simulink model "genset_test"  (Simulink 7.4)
settings: Solver=ode23t  StartTime=0.0  StopTime=10  RelTol=1e-4
undefined symbols (not defined in the file or in its folder): bits, D1, Delta
libraries: powerlib x25, powerlib_extras x3, dspswit3 x1

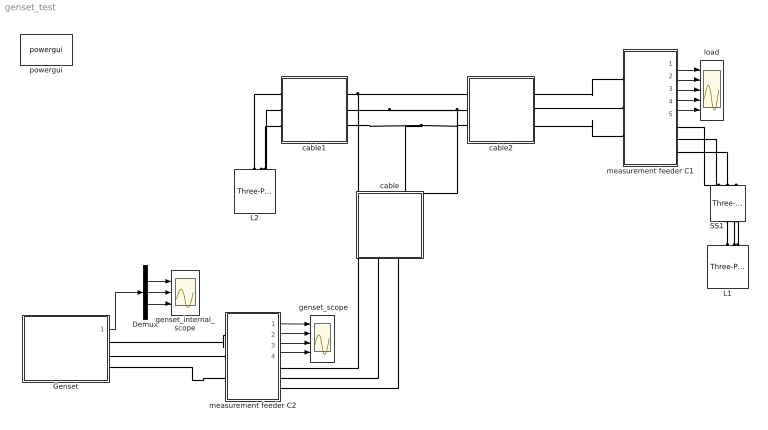
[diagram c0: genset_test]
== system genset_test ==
  " genset_scope" : Scope  NumInputPorts=4
  Demux : Demux  Outputs=3
  Genset : Subsystem
  L1 : powerlib/Elements/Three-Phase Series RLC Load  DialogController=POWERSYS.PowerSysDialog  PhysicalDomain=powersysdomain  SubClassName=unknown  LeftPortType=p1  RightPortType=p1  LConnTagsString=A|B|C  Configuration=Y (grounded)  NominalVoltage=208  NominalFrequency=60  ActivePower=4000  InductivePower=0  CapacitivePower=0  Measurements=None
  L2 : powerlib/Elements/Three-Phase Series RLC Load  DialogController=POWERSYS.PowerSysDialog  PhysicalDomain=powersysdomain  SubClassName=unknown  LeftPortType=p1  RightPortType=p1  LConnTagsString=A|B|C  Configuration=Y (grounded)  NominalVoltage=208  NominalFrequency=60  ActivePower=1897  InductivePower=0  CapacitivePower=0  Measurements=None
  SS1 : powerlib/Elements/Three-Phase Breaker  DialogController=POWERSYS.PowerSysDialog  SystemSampleTime=-1  InitialState=open  SwitchA=on  SwitchB=on  SwitchC=on  SwitchTimes=[3+1/5 7]  External=off  BreakerResistance=.00001  SnubberResistance=1e10  SnubberCapacitance=inf  Measurements=None
  cable : Subsystem  mask{R=.0656, L=.0021, C=345.6}
  cable1 : Subsystem  mask{R=.002657, L=.000641, C=2020}
  cable2 : Subsystem  mask{R=0.0168, L=0.00407, C=336}
  genset_internal_scope : Scope  NumInputPorts=3
  load : Scope  NumInputPorts=5
  measurement feeder C1 : Subsystem
  measurement feeder C2 : Subsystem
  powergui : powerlib/powergui  Priority=1  SystemSampleTime=-1  SimulationMode=Discrete  SampleTime=20e-6  frequency=60  SPID=off  DisableSnubberDevices=off  DisableRonSwitches=off  DisableVfSwitches=off  SwTol=0  Interpol=off  frequencyindice=60  echomessages=off  HookPort=off  DisplayEquations=off  FunctionMessages=off  EnableUseOfTLC=off  x0status=blocks  RestoreLinks=warning  Frange=[0:2:500]  Ylog=off  Xlog=on  ShowGrid=off  save=off  variable=ZData  ZoomFFT=on  StartTime=0.0  cycles=1  DisplayStyle=1  fundamental=60  FreqAxis=off  MaxFrequency=1000  frequencyindicesteady=1  RmsSteady=1  display=off  Ts=0  methode=off
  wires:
  measurement feeder C2/1(Vabc) -> " genset_scope"/1
  measurement feeder C2/2(Iabc) -> " genset_scope"/2
  measurement feeder C2/3(PQ) -> " genset_scope"/3
  measurement feeder C2/4(RMS (V-I)) -> " genset_scope"/4
  measurement feeder C1/5(w) -> load/5
  measurement feeder C1/4(RMS (V-I)) -> load/4
  measurement feeder C1/3(PQ) -> load/3
  measurement feeder C1/2(Iabc) -> load/2
  measurement feeder C1/1(Vabc) -> load/1
  Demux/3 -> genset_internal_scope/3
  Demux/2 -> genset_internal_scope/2
  Demux/1 -> genset_internal_scope/1
  Genset/1(m) -> Demux/1
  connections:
  cable1/RConn2 -- L2/LConn2
  measurement feeder C1/RConn1 -- SS1/LConn1
  measurement feeder C1/RConn2 -- SS1/LConn2
  measurement feeder C1/RConn3 -- SS1/LConn3
  L1/LConn1 -- SS1/RConn1
  L1/LConn2 -- SS1/RConn2
  L1/LConn3 -- SS1/RConn3
  cable1/LConn1 -- cable/RConn1 -- cable2/RConn1
  cable2/RConn2 -- cable/RConn2 -- cable1/LConn2
  cable2/RConn3 -- cable1/LConn3 -- cable/RConn3
  cable2/LConn2 -- measurement feeder C1/LConn2
  measurement feeder C2/LConn1 -- Genset/RConn1
  Genset/RConn3 -- measurement feeder C2/LConn3
  measurement feeder C2/RConn1 -- cable/LConn1
  measurement feeder C2/RConn2 -- cable/LConn2
  measurement feeder C2/RConn3 -- cable/LConn3
  cable1/RConn1 -- L2/LConn1
  L2/LConn3 -- cable1/RConn3
  measurement feeder C1/LConn1 -- cable2/LConn1
  measurement feeder C1/LConn3 -- cable2/LConn3
  Genset/RConn2 -- measurement feeder C2/LConn2

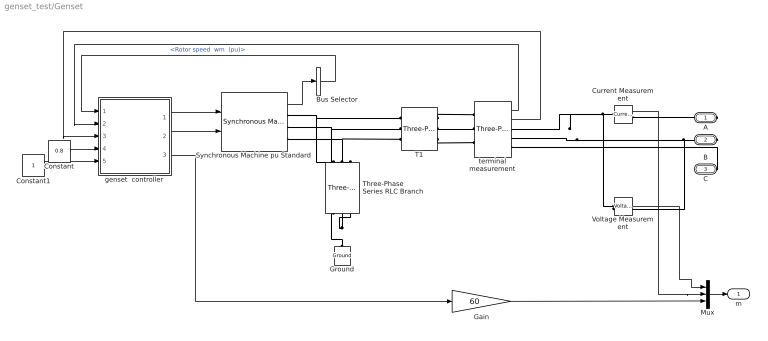
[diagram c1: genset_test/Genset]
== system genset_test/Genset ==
  Bus Selector : BusSelector  OutputSignals="Mechanical.Rotor speed  wm  (pu)"
  Constant : Constant  Value=0.8  OutDataType=fixdt(1, 16)  OutScaling=2^0
  Constant1 : Constant  OutDataType=fixdt(1, 16)  OutScaling=2^0
  Current Measurement : powerlib/Measurements/Current Measurement  DialogController=POWERSYS.PowerSysDialog  SystemSampleTime=-1  PhasorSimulation=off  OutputType=Complex  PSBequivalent=0
  Gain : Gain  Gain=60  ParameterDataType=fixdt(1, 16)  ParameterScaling=2^0  OutDataType=fixdt(1, 16)  OutScaling=2^0
  Ground : powerlib/Elements/Ground  DialogController=POWERSYS.PowerSysDialog  PhysicalDomain=powersysdomain  SubClassName=unknown  LeftPortType=p1  RightPortType=p1  LConnTagsString=a
  Mux : Mux  Inputs=3
  Synchronous Machine pu Standard : powerlib/Machines/Synchronous Machine pu Standard  DialogController=POWERSYS.PowerSysDialog  SystemSampleTime=-1  PresetModel=No  MechanicalLoad=Mechanical power Pm  ShowDetailedParameters=on  RotorType=Salient-pole  NominalParameters="[ 16000  240   60]"  Reactances1=[ 1.81, 0.3, 0.23, 1.76, 0.65, 0.25, 0.15 ]  Reactances2="[ 1.204, 0.125, 0.056, 0.533,  0.051,  0.037 ]"  dAxisTimeConstants=Short-circuit  qAxisTimeConstants=Short-circuit  TimeConstants1="[ 4.4849  0.0681  0.1  ]"  TimeConstants2=[ 8.0, 0.03, 1.0, 0.07 ]  TimeConstants3="[  .35523  0.00015  0.067  ]"  TimeConstants4=[ 8.0, 0.03, 0.3371, 0.0295 ]  TimeConstants5=[ 1.01, 0.053, 0.1 ]  TimeConstants6=[ 1.3201, 0.023, 1.0, 0.07 ]  TimeConstants7=[0.35523 0.00015 0.0067]  TimeConstants8=[ 1.3201, 0.0231, 0.3371, 0.0295 ]  StatorResistance=0.0217  Mechanical=[ .19 0 2 ]  PolePairs=2  InitialConditions="[ 0  0  0  0  0  0  0  0  1 ]"  SetSaturation=off  Saturation=[0.6404,0.7127,0.8441,0.9214,0.9956,1.082,1.19,1.316,1.457;0.7,0.7698,0.8872,0.9466,0.9969,1.046,1.1,1.151,1.201]  Units=per unit standard parameters  LoadFlowParameters=[1 0 0 0 0]  TsPowergui=0  TsBlock=-1  IterativeModel=Forward Euler
  T1 : powerlib/Elements/Three-Phase Transformer (Two Windings)  DialogController=POWERSYS.PowerSysDialog  SystemSampleTime=-1  Winding1Connection=Delta (D1)  UNITS=SI  NominalPower=[ 45e3 , 60 ]  Winding1=[240 .02688 .10752/(2*pi*60)]  Winding2Connection=Yg  Winding2=[208 .005047 .201899/(2*pi*60)]  SetSaturation=off  Rm=1e+08  Lm=7650.8  Saturation=[0 0;1359.8 0.93633;5.6659e+05 1.186]  Hysteresis=off  DataFile='hysteresis'  SetInitialFlux=off  InitialFluxes=[0.62422 -0.62422 0.54618]  Measurements=None  MoreParameters=off  BreakLoop=off  DataType=on  TransfoNumber=1
  Three-Phase Series RLC Branch : powerlib/Elements/Three-Phase Series RLC Branch  DialogController=POWERSYS.PowerSysDialog  PhysicalDomain=powersysdomain  SubClassName=unknown  LeftPortType=p1  RightPortType=p1  LConnTagsString=A|B|C  RConnTagsString=A|B|C  BranchType=C  Resistance=1  Inductance=1e-3  Capacitance=1.e-4  Measurements=None
  Voltage Measurement : powerlib/Measurements/Voltage Measurement  DialogController=POWERSYS.PowerSysDialog  SystemSampleTime=-1  PhasorSimulation=off  OutputType=Complex  PSBequivalent=0
  genset  controller : Subsystem  mask{Vbase=208, Sbase=12500}
  terminal measurement : powerlib/Measurements/Three-Phase V-I Measurement  DialogController=POWERSYS.PowerSysDialog  SystemSampleTime=-1  VoltageMeasurement=phase-to-ground  SetLabelV=off  LabelV=Vabc  Vpu=off  CurrentMeasurement=yes  SetLabelI=off  LabelI=Iabc  Ipu=off  Pbase=100e6  Vbase=500e3  OutputType=Complex  PhasorSimulation=off  PSBequivalent=0
  A : PMIOPort  Port=1  Side=Right
  B : PMIOPort  Port=2  Side=Right
  C : PMIOPort  Port=3  Side=Right
  m : Outport
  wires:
  Synchronous Machine pu Standard/1 -> Bus Selector/1
  terminal measurement/1 -> genset  controller/2(Vabc)
  terminal measurement/2 -> genset  controller/3(Iabc)
  Constant1/1 -> genset  controller/5(Ereq1)
  genset  controller/1(Pmech) -> Synchronous Machine pu Standard/1
  genset  controller/2(Vf) -> Synchronous Machine pu Standard/2
  Voltage Measurement/1 -> Mux/1
  Current Measurement/1 -> Mux/2
  Constant/1 -> genset  controller/4(Preq)
  Gain/1 -> Mux/3
  genset  controller/3(w) -> Gain/1
  Bus Selector/1 -> genset  controller/1(wr)  "<Rotor speed  wm  (pu)>"
  Mux/1 -> m/1
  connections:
  Current Measurement/LConn1 -- terminal measurement/RConn1 -- Voltage Measurement/LConn1
  Ground/LConn1 -- Three-Phase Series RLC Branch/RConn2 -- Three-Phase Series RLC Branch/RConn3 -- Three-Phase Series RLC Branch/RConn1
  Synchronous Machine pu Standard/RConn1 -- Three-Phase Series RLC Branch/LConn1 -- T1/LConn1
  Synchronous Machine pu Standard/RConn2 -- Three-Phase Series RLC Branch/LConn2 -- T1/LConn2
  Synchronous Machine pu Standard/RConn3 -- Three-Phase Series RLC Branch/LConn3 -- T1/LConn3
  T1/RConn1 -- terminal measurement/LConn1
  T1/RConn2 -- terminal measurement/LConn2
  T1/RConn3 -- terminal measurement/LConn3
  B/RConn1 -- terminal measurement/RConn2 -- Voltage Measurement/LConn2
  A/RConn1 -- Current Measurement/RConn1
  C/RConn1 -- terminal measurement/RConn3

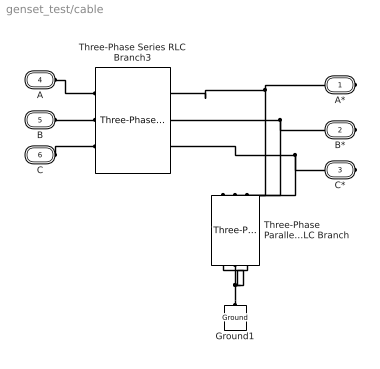
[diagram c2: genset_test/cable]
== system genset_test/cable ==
  Ground1 : powerlib/Elements/Ground  DialogController=POWERSYS.PowerSysDialog  PhysicalDomain=powersysdomain  SubClassName=unknown  LeftPortType=p1  RightPortType=p1  LConnTagsString=a
  Three-Phase Parallel RLC Branch : powerlib/Elements/Three-Phase Parallel RLC Branch  DialogController=POWERSYS.PowerSysDialog  PhysicalDomain=powersysdomain  SubClassName=unknown  LeftPortType=p1  RightPortType=p1  LConnTagsString=A|B|C  RConnTagsString=A|B|C  BranchType=C  Resistance=1  Inductance=1e-3  Capacitance=1/(C*2*pi*60)  Measurements=None
  Three-Phase Series RLC Branch3 : powerlib/Elements/Three-Phase Series RLC Branch  DialogController=POWERSYS.PowerSysDialog  PhysicalDomain=powersysdomain  SubClassName=unknown  LeftPortType=p1  RightPortType=p1  LConnTagsString=A|B|C  RConnTagsString=A|B|C  BranchType=RL  Resistance=R  Inductance=L/(2*pi*60)  Capacitance=1/(336*2*pi*60)  Measurements=None
  A* : PMIOPort  Tag=PMCPort  Port=1  Side=Right
  B* : PMIOPort  Tag=PMCPort  Port=2  Side=Right
  C* : PMIOPort  Tag=PMCPort  Port=3  Side=Right
  A : PMIOPort  Tag=PMCPort  Port=4  Side=Left
  B : PMIOPort  Tag=PMCPort  Port=5  Side=Left
  C : PMIOPort  Tag=PMCPort  Port=6  Side=Left
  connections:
  Ground1/LConn1 -- Three-Phase Parallel RLC Branch/RConn2 -- Three-Phase Parallel RLC Branch/RConn3 -- Three-Phase Parallel RLC Branch/RConn1
  A*/RConn1 -- Three-Phase Series RLC Branch3/LConn1 -- Three-Phase Parallel RLC Branch/LConn1
  B*/RConn1 -- Three-Phase Series RLC Branch3/LConn2 -- Three-Phase Parallel RLC Branch/LConn2
  C*/RConn1 -- Three-Phase Series RLC Branch3/LConn3 -- Three-Phase Parallel RLC Branch/LConn3
  A/RConn1 -- Three-Phase Series RLC Branch3/RConn1
  B/RConn1 -- Three-Phase Series RLC Branch3/RConn2
  C/RConn1 -- Three-Phase Series RLC Branch3/RConn3

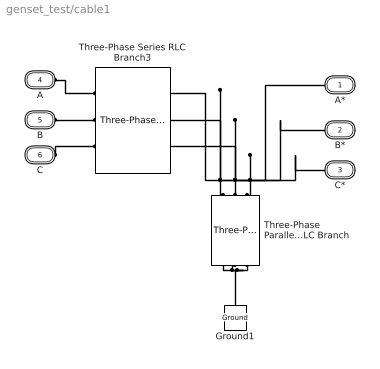
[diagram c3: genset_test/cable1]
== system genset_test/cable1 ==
  Ground1 : powerlib/Elements/Ground  DialogController=POWERSYS.PowerSysDialog  PhysicalDomain=powersysdomain  SubClassName=unknown  LeftPortType=p1  RightPortType=p1  LConnTagsString=a
  Three-Phase Parallel RLC Branch : powerlib/Elements/Three-Phase Parallel RLC Branch  DialogController=POWERSYS.PowerSysDialog  PhysicalDomain=powersysdomain  SubClassName=unknown  LeftPortType=p1  RightPortType=p1  LConnTagsString=A|B|C  RConnTagsString=A|B|C  BranchType=C  Resistance=1  Inductance=1e-3  Capacitance=1/(C*2*pi*60)  Measurements=None
  Three-Phase Series RLC Branch3 : powerlib/Elements/Three-Phase Series RLC Branch  DialogController=POWERSYS.PowerSysDialog  PhysicalDomain=powersysdomain  SubClassName=unknown  LeftPortType=p1  RightPortType=p1  LConnTagsString=A|B|C  RConnTagsString=A|B|C  BranchType=RL  Resistance=R  Inductance=L/(2*pi*60)  Capacitance=1/(336*2*pi*60)  Measurements=None
  A* : PMIOPort  Tag=PMCPort  Port=1  Side=Right
  B* : PMIOPort  Tag=PMCPort  Port=2  Side=Right
  C* : PMIOPort  Tag=PMCPort  Port=3  Side=Right
  A : PMIOPort  Tag=PMCPort  Port=4  Side=Left
  B : PMIOPort  Tag=PMCPort  Port=5  Side=Left
  C : PMIOPort  Tag=PMCPort  Port=6  Side=Left
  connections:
  Three-Phase Parallel RLC Branch/RConn3 -- Ground1/LConn1 -- Three-Phase Parallel RLC Branch/RConn2 -- Three-Phase Parallel RLC Branch/RConn1
  Three-Phase Parallel RLC Branch/LConn1 -- A*/RConn1 -- Three-Phase Series RLC Branch3/LConn1
  Three-Phase Parallel RLC Branch/LConn2 -- B*/RConn1 -- Three-Phase Series RLC Branch3/LConn2
  Three-Phase Parallel RLC Branch/LConn3 -- C*/RConn1 -- Three-Phase Series RLC Branch3/LConn3
  A/RConn1 -- Three-Phase Series RLC Branch3/RConn1
  B/RConn1 -- Three-Phase Series RLC Branch3/RConn2
  C/RConn1 -- Three-Phase Series RLC Branch3/RConn3

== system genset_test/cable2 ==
  Ground1 : powerlib/Elements/Ground  DialogController=POWERSYS.PowerSysDialog  PhysicalDomain=powersysdomain  SubClassName=unknown  LeftPortType=p1  RightPortType=p1  LConnTagsString=a
  Three-Phase Parallel RLC Branch : powerlib/Elements/Three-Phase Parallel RLC Branch  DialogController=POWERSYS.PowerSysDialog  PhysicalDomain=powersysdomain  SubClassName=unknown  LeftPortType=p1  RightPortType=p1  LConnTagsString=A|B|C  RConnTagsString=A|B|C  BranchType=C  Resistance=1  Inductance=1e-3  Capacitance=1/(C*2*pi*60)  Measurements=None
  Three-Phase Series RLC Branch3 : powerlib/Elements/Three-Phase Series RLC Branch  DialogController=POWERSYS.PowerSysDialog  PhysicalDomain=powersysdomain  SubClassName=unknown  LeftPortType=p1  RightPortType=p1  LConnTagsString=A|B|C  RConnTagsString=A|B|C  BranchType=RL  Resistance=R  Inductance=L/(2*pi*60)  Capacitance=1/(336*2*pi*60)  Measurements=None
  A* : PMIOPort  Tag=PMCPort  Port=1  Side=Right
  B* : PMIOPort  Tag=PMCPort  Port=2  Side=Right
  C* : PMIOPort  Tag=PMCPort  Port=3  Side=Right
  A : PMIOPort  Tag=PMCPort  Port=4  Side=Left
  B : PMIOPort  Tag=PMCPort  Port=5  Side=Left
  C : PMIOPort  Tag=PMCPort  Port=6  Side=Left
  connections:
  Three-Phase Parallel RLC Branch/RConn3 -- Ground1/LConn1 -- Three-Phase Parallel RLC Branch/RConn2 -- Three-Phase Parallel RLC Branch/RConn1
  Three-Phase Parallel RLC Branch/LConn1 -- A*/RConn1 -- Three-Phase Series RLC Branch3/LConn1
  Three-Phase Parallel RLC Branch/LConn2 -- B*/RConn1 -- Three-Phase Series RLC Branch3/LConn2
  Three-Phase Parallel RLC Branch/LConn3 -- C*/RConn1 -- Three-Phase Series RLC Branch3/LConn3
  A/RConn1 -- Three-Phase Series RLC Branch3/RConn1
  B/RConn1 -- Three-Phase Series RLC Branch3/RConn2
  C/RConn1 -- Three-Phase Series RLC Branch3/RConn3

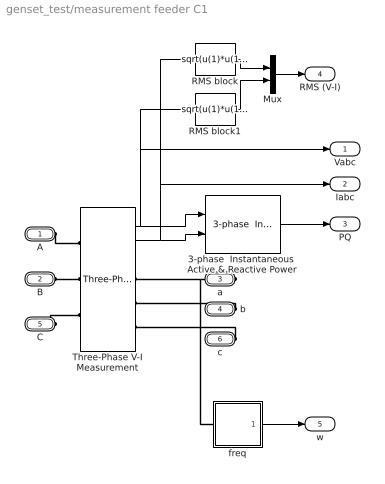
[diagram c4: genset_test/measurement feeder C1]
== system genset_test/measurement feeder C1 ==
  3-phase  Instantaneous  Active & Reactive Power : powerlib_extras/Measurements/3-phase  Instantaneous  Active & Reactive Power  DialogController=POWERSYS.PowerSysDialog  SystemSampleTime=-1
  Mux : Mux  Inputs=2
  RMS block : Fcn  Expr=sqrt(u(1)*u(1)+u(2)*u(2)+u(3)*u(3))/sqrt(3)
  RMS block1 : Fcn  Expr=sqrt(u(1)*u(1)+u(2)*u(2)+u(3)*u(3))/sqrt(3)
  Three-Phase V-I Measurement : powerlib/Measurements/Three-Phase V-I Measurement  DialogController=POWERSYS.PowerSysDialog  SystemSampleTime=-1  VoltageMeasurement=phase-to-ground  SetLabelV=off  LabelV=Vabc  Vpu=off  CurrentMeasurement=yes  SetLabelI=off  LabelI=Iabc  Ipu=off  Pbase=100e6  Vbase=500e3  OutputType=Complex  PhasorSimulation=off  PSBequivalent=0
  freq : Subsystem  AncestorBlock=|
      | UWM_blocks/frequency
      | measurement
      | (zero-crossings)
  A : PMIOPort  Port=1  Side=Left
  B : PMIOPort  Port=2  Side=Left
  a : PMIOPort  Port=3  Side=Right
  b : PMIOPort  Port=4  Side=Right
  C : PMIOPort  Port=5  Side=Left
  c : PMIOPort  Port=6  Side=Right
  Vabc : Outport  OutDataType=fixdt(1, 16)  OutScaling=2^0
  Iabc : Outport  Port=2  OutDataType=fixdt(1, 16)  OutScaling=2^0
  PQ : Outport  Port=3  OutDataType=fixdt(1, 16)  OutScaling=2^0
  RMS (V-I) : Outport  Port=4  OutDataType=fixdt(1, 16)  OutScaling=2^0
  w : Outport  Port=5  OutDataType=fixdt(1, 16)  OutScaling=2^0
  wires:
  Three-Phase V-I Measurement/1 -> Vabc/1, RMS block1/1, 3-phase  Instantaneous  Active & Reactive Power/1
  Three-Phase V-I Measurement/2 -> Iabc/1, RMS block/1, 3-phase  Instantaneous  Active & Reactive Power/2
  Mux/1 -> RMS (V-I)/1
  RMS block/1 -> Mux/1
  RMS block1/1 -> Mux/2
  3-phase  Instantaneous  Active & Reactive Power/1 -> PQ/1
  freq/1(w (Hz)) -> w/1
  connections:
  c/RConn1 -- Three-Phase V-I Measurement/RConn3
  C/RConn1 -- Three-Phase V-I Measurement/LConn3
  b/RConn1 -- Three-Phase V-I Measurement/RConn2
  a/RConn1 -- Three-Phase V-I Measurement/RConn1 -- freq/LConn1
  B/RConn1 -- Three-Phase V-I Measurement/LConn2
  A/RConn1 -- Three-Phase V-I Measurement/LConn1

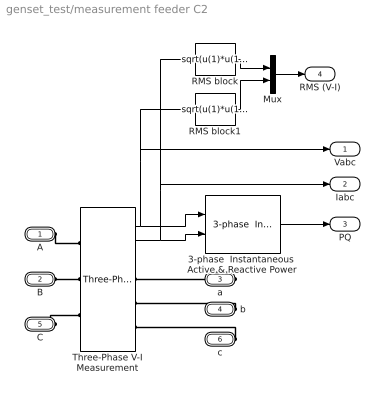
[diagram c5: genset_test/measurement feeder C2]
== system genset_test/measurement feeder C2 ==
  3-phase  Instantaneous  Active & Reactive Power : powerlib_extras/Measurements/3-phase  Instantaneous  Active & Reactive Power  DialogController=POWERSYS.PowerSysDialog  SystemSampleTime=-1
  Mux : Mux  Inputs=2
  RMS block : Fcn  Expr=sqrt(u(1)*u(1)+u(2)*u(2)+u(3)*u(3))/sqrt(3)
  RMS block1 : Fcn  Expr=sqrt(u(1)*u(1)+u(2)*u(2)+u(3)*u(3))/sqrt(3)
  Three-Phase V-I Measurement : powerlib/Measurements/Three-Phase V-I Measurement  DialogController=POWERSYS.PowerSysDialog  SystemSampleTime=-1  VoltageMeasurement=phase-to-ground  SetLabelV=off  LabelV=Vabc  Vpu=off  CurrentMeasurement=yes  SetLabelI=off  LabelI=Iabc  Ipu=off  Pbase=100e6  Vbase=500e3  OutputType=Complex  PhasorSimulation=off  PSBequivalent=0
  A : PMIOPort  Port=1  Side=Left
  B : PMIOPort  Port=2  Side=Left
  a : PMIOPort  Port=3  Side=Right
  b : PMIOPort  Port=4  Side=Right
  C : PMIOPort  Port=5  Side=Left
  c : PMIOPort  Port=6  Side=Right
  Vabc : Outport  OutDataType=fixdt(1, 16)  OutScaling=2^0
  Iabc : Outport  Port=2  OutDataType=fixdt(1, 16)  OutScaling=2^0
  PQ : Outport  Port=3  OutDataType=fixdt(1, 16)  OutScaling=2^0
  RMS (V-I) : Outport  Port=4  OutDataType=fixdt(1, 16)  OutScaling=2^0
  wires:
  Three-Phase V-I Measurement/1 -> Vabc/1, RMS block1/1, 3-phase  Instantaneous  Active & Reactive Power/1
  Three-Phase V-I Measurement/2 -> Iabc/1, RMS block/1, 3-phase  Instantaneous  Active & Reactive Power/2
  Mux/1 -> RMS (V-I)/1
  RMS block/1 -> Mux/1
  RMS block1/1 -> Mux/2
  3-phase  Instantaneous  Active & Reactive Power/1 -> PQ/1
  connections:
  c/RConn1 -- Three-Phase V-I Measurement/RConn3
  C/RConn1 -- Three-Phase V-I Measurement/LConn3
  b/RConn1 -- Three-Phase V-I Measurement/RConn2
  a/RConn1 -- Three-Phase V-I Measurement/RConn1
  B/RConn1 -- Three-Phase V-I Measurement/LConn2
  A/RConn1 -- Three-Phase V-I Measurement/LConn1

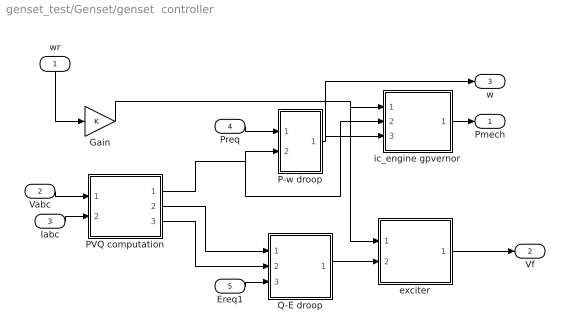
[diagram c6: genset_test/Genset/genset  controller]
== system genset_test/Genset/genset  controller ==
  wr : Inport
  Vabc : Inport  Port=2
  Iabc : Inport  Port=3
  Preq : Inport  Port=4
  Ereq1 : Inport  Port=5
  Gain : Gain  ParameterDataType=fixdt(1, 16)  ParameterScaling=2^0  OutDataType=fixdt(1, 16)  OutScaling=2^0
  P-w droop : Subsystem
  PVQ computation : Subsystem
  Q-E droop : Subsystem
  exciter : Subsystem
  ic_engine gpvernor : Subsystem
  Pmech : Outport
  Vf : Outport  Port=2
  w : Outport  Port=3
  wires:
  P-w droop/1(w) -> w/1, ic_engine gpvernor/3(w)
  PVQ computation/1(P_pu) -> P-w droop/2(P), ic_engine gpvernor/2(Pmeas)
  PVQ computation/3(Q_pu) -> Q-E droop/2(Q)
  Q-E droop/1(Vpk) -> exciter/2(Ef_mcd_wr)
  ic_engine gpvernor/1(Pmech) -> Pmech/1
  Vabc/1 -> PVQ computation/1(Vabc)
  Iabc/1 -> PVQ computation/2(Iabc)
  exciter/1(Ef) -> Vf/1
  Preq/1 -> P-w droop/1(P_req)
  Ereq1/1 -> Q-E droop/3(E_req)
  PVQ computation/2(Vt) -> Q-E droop/1(v_meas)
  Gain/1 -> ic_engine gpvernor/1(wr), exciter/1(wr)
  wr/1 -> Gain/1

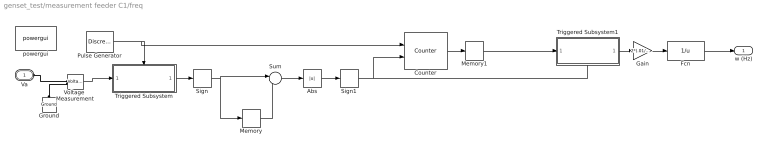
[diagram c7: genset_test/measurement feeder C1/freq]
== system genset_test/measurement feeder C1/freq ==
  Abs : Abs  OutDataType=fixdt(1, 16)  OutScaling=2^0
  Counter : dspswit3/Counter  Direction=Up  CountEvent=Rising edge  CounterSize=32 bits  MaxCount=255  InitialCount=0  Output=Count  HitValue=32  ResetInput=on  SamplesPerFrame=1  Ts=1  CntDtype=double  HitDtype=Logical
  Fcn : Fcn  Expr=1/u
  Gain : Gain  Gain=2*(.01/60)  ParameterDataType=fixdt(1, 16)  ParameterScaling=2^0  OutDataType=fixdt(1, 16)  OutScaling=2^0
  Ground : powerlib/Elements/Ground  DialogController=POWERSYS.PowerSysDialog  PhysicalDomain=powersysdomain  SubClassName=unknown  LeftPortType=p1  RightPortType=p1  LConnTagsString=a
  Memory : Memory
  Memory1 : Memory  InheritSampleTime=on
  Pulse Generator : DiscretePulseGenerator  PulseType=Time based  Amplitude=1  Period=.01/60  PulseWidth=50  PhaseDelay=0  SampleTime=1
  Sign : Signum
  Sign1 : Signum
  Sum : Sum  Inputs=|+-  OutDataType=fixdt(1, 16)  OutScaling=2^0
  Triggered Subsystem : Subsystem  TreatAsAtomicUnit=on
  Triggered Subsystem1 : Subsystem  TreatAsAtomicUnit=on
  Voltage  Measurement : powerlib/Measurements/Voltage Measurement  DialogController=POWERSYS.PowerSysDialog  SystemSampleTime=-1  PhasorSimulation=off  OutputType=Complex  PSBequivalent=0
  powergui : powerlib/powergui  Priority=1  SystemSampleTime=-1  SimulationMode=Continuous  SampleTime=50e-6  frequency=60  SPID=off  DisableSnubberDevices=off  DisableRonSwitches=off  DisableVfSwitches=off  SwTol=0  Interpol=off  frequencyindice=0  echomessages=off  HookPort=off  DisplayEquations=off  FunctionMessages=off  EnableUseOfTLC=off  x0status=blocks  RestoreLinks=warning  Frange=[0:2:500]  Ylog=off  Xlog=on  ShowGrid=off  save=off  variable=ZData  ZoomFFT=on  StartTime=0.0  cycles=1  DisplayStyle=1  fundamental=60  FreqAxis=off  MaxFrequency=1000  frequencyindicesteady=1  RmsSteady=1  display=off  Ts=0  methode=off
  Va : PMIOPort  Tag=PMCPort  Port=1  Side=Left
  w (Hz) : Outport
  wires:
  Pulse Generator/1 -> Triggered Subsystem/Trigger, Counter/1
  Triggered Subsystem/1(Out1) -> Sign/1
  Sign/1 -> Sum/1, Memory/1
  Memory/1 -> Sum/2
  Sum/1 -> Abs/1
  Abs/1 -> Sign1/1
  Sign1/1 -> Counter/2, Triggered Subsystem1/Trigger
  Triggered Subsystem1/1(Out1) -> Gain/1
  Gain/1 -> Fcn/1
  Counter/1 -> Memory1/1
  Memory1/1 -> Triggered Subsystem1/1(In1)
  Voltage  Measurement/1 -> Triggered Subsystem/1(In1)
  Fcn/1 -> w (Hz)/1
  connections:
  Ground/LConn1 -- Voltage  Measurement/LConn2
  Va/RConn1 -- Voltage  Measurement/LConn1

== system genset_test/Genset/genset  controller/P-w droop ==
  note: P
  P_req : Inport
  P : Inport  Port=2
  Sum2 : Sum  Inputs=+-|  OutDataType=sfix(16)  OutScaling=2^0
  Sum3 : Sum  Inputs=+++  OutDataType=sfix(16)  OutScaling=2^0
  limiter : Subsystem
  mP droop : Gain  Gain=pi  ParameterDataType=sfix(16)  ParameterScaling=2^0  OutDataType=sfix(16)  OutScaling=2^0
  rad2pu : Gain  Gain=1/(2*pi*60)  ParameterDataType=sfix(16)  ParameterScaling=2^0  OutDataType=sfix(16)  OutScaling=2^0
  w0 : Constant  Value=60*2*pi  OutDataType=fixdt(1, 16)  OutScaling=2^0
  w : Outport
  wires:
  P_req/1 -> Sum2/1
  mP droop/1 -> Sum3/2
  limiter/1(Out1) -> Sum3/1
  w0/1 -> Sum3/3
  Sum2/1 -> mP droop/1
  P/1 -> limiter/1(In1), Sum2/2
  Sum3/1 -> rad2pu/1
  rad2pu/1 -> w/1

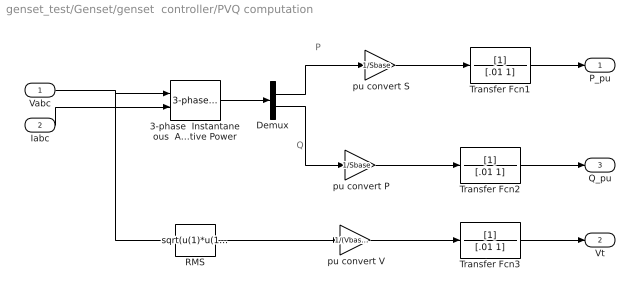
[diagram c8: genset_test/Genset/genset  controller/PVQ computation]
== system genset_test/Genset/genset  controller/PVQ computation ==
  note: P
  note: Q
  Vabc : Inport  OutDataType=fixdt(1, 16)  OutScaling=2^0
  Iabc : Inport  Port=2  OutDataType=fixdt(1, 16)  OutScaling=2^0
  " pu convert P" : Gain  Gain=1/Sbase  ParameterDataType=sfix(16)  ParameterScaling=2^0  OutDataType=sfix(16)  OutScaling=2^0
  " pu convert S" : Gain  Gain=1/Sbase  ParameterDataType=sfix(16)  ParameterScaling=2^0  OutDataType=sfix(16)  OutScaling=2^0
  " pu convert V" : Gain  Gain=1/(Vbase/sqrt(3))  ParameterDataType=sfix(16)  ParameterScaling=2^0  OutDataType=sfix(16)  OutScaling=2^0
  3-phase  Instantaneous  Active & Reactive Power : powerlib_extras/Measurements/3-phase  Instantaneous  Active & Reactive Power  DialogController=POWERSYS.PowerSysDialog  SystemSampleTime=-1
  Demux : Demux  Outputs=2
  RMS : Fcn  Expr=sqrt(u(1)*u(1)+u(2)*u(2)+u(3)*u(3))/sqrt(3)
  Transfer Fcn1 : TransferFcn  Denominator=[.01 1]
  Transfer Fcn2 : TransferFcn  Denominator=[.01 1]
  Transfer Fcn3 : TransferFcn  Denominator=[.01 1]
  P_pu : Outport  OutDataType=fixdt(1, 16)  OutScaling=2^0
  Vt : Outport  Port=2  OutDataType=fixdt(1, 16)  OutScaling=2^0
  Q_pu : Outport  Port=3  OutDataType=fixdt(1, 16)  OutScaling=2^0
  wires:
  Iabc/1 -> 3-phase  Instantaneous  Active & Reactive Power/2
  RMS/1 -> " pu convert V"/1
  Demux/2 -> " pu convert P"/1
  Demux/1 -> " pu convert S"/1
  3-phase  Instantaneous  Active & Reactive Power/1 -> Demux/1
  Vabc/1 -> RMS/1, 3-phase  Instantaneous  Active & Reactive Power/1
  Transfer Fcn1/1 -> P_pu/1
  " pu convert S"/1 -> Transfer Fcn1/1
  Transfer Fcn2/1 -> Q_pu/1
  " pu convert P"/1 -> Transfer Fcn2/1
  Transfer Fcn3/1 -> Vt/1
  " pu convert V"/1 -> Transfer Fcn3/1

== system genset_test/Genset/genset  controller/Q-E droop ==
  note: Q
  v_meas : Inport
  Q : Inport  Port=2
  E_req : Inport  Port=3
  PI-Control : Subsystem
  Sum : Sum  Inputs=|-+  OutDataType=sfix(16)  OutScaling=2^0
  Sum1 : Sum  Inputs=|+-  OutDataType=sfix(16)  OutScaling=2^0
  "mQ droop " : Gain  Gain=0.05  ParameterDataType=sfix(16)  ParameterScaling=2^0  OutDataType=sfix(16)  OutScaling=2^0
  Vpk : Outport
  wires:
  Sum1/1 -> PI-Control/1(In1)
  Sum/1 -> Sum1/1
  "mQ droop "/1 -> Sum/1
  PI-Control/1(Out1) -> Vpk/1
  Q/1 -> "mQ droop "/1
  E_req/1 -> Sum/2
  v_meas/1 -> Sum1/2

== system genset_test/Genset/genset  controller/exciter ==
  wr : Inport  OutDataType=fixdt(1, 16)  OutScaling=2^0
  Ef_mcd_wr : Inport  Port=2  OutDataType=fixdt(1, 16)  OutScaling=2^0
  Product : Product  OutDataType=fixdt(1, 16)  OutScaling=2^0
  Saturation : Saturate  UpperLimit=10  LowerLimit=-10  OutDataType=fixdt(1, 16)  OutScaling=2^0
  Transfer Fcn : TransferFcn  Denominator=[.001 1]
  Ef : Outport  OutDataType=fixdt(1, 16)  OutScaling=2^0
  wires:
  wr/1 -> Product/2
  Ef_mcd_wr/1 -> Product/1
  Product/1 -> Saturation/1
  Saturation/1 -> Transfer Fcn/1
  Transfer Fcn/1 -> Ef/1

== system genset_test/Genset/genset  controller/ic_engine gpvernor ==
  wr : Inport  OutDataType=fixdt(1, 16)  OutScaling=2^0
  Pmeas : Inport  Port=2  OutDataType=fixdt(1, 16)  OutScaling=2^0
  w : Inport  Port=3  OutDataType=fixdt(1, 16)  OutScaling=2^0
  IC_engine : Subsystem
  governor : Subsystem
  Pmech : Outport  OutDataType=fixdt(1, 16)  OutScaling=2^0
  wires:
  governor/1(fuel_cmd) -> IC_engine/1(fuel_cmd)
  Pmeas/1 -> governor/1(Pmeas)
  IC_engine/1(Pmech) -> Pmech/1
  wr/1 -> governor/3(wr), IC_engine/2(wr)
  w/1 -> governor/2(w)

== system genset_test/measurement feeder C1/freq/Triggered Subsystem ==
  In1 : Inport  OutDataType=fixdt(1, 16)  OutScaling=2^0
  Trigger : TriggerPort
  Out1 : Outport  OutDataType=fixdt(1, 16)  OutScaling=2^0
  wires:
  In1/1 -> Out1/1

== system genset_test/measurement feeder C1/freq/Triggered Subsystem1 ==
  In1 : Inport  OutDataType=fixdt(1, 16)  OutScaling=2^0
  Trigger : TriggerPort
  Out1 : Outport  OutDataType=fixdt(1, 16)  OutScaling=2^0
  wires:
  In1/1 -> Out1/1

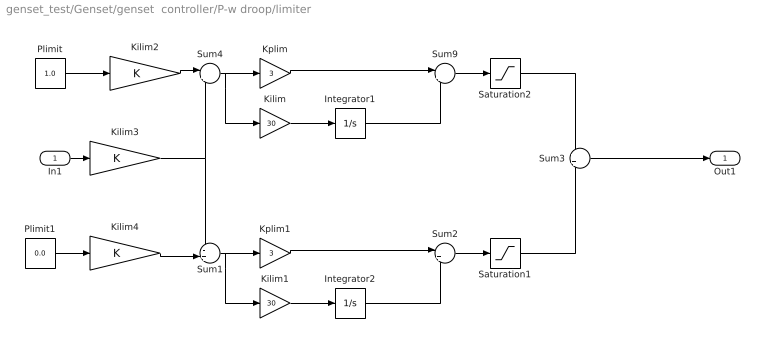
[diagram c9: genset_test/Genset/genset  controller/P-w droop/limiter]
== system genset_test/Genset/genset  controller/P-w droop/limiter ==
  In1 : Inport
  Integrator1 : Integrator  UpperSaturationLimit=0  LowerSaturationLimit=-2*pi
  Integrator2 : Integrator  UpperSaturationLimit=2*pi  LowerSaturationLimit=0
  Kilim : Gain  Gain=30  ParameterDataType=sfix(16)  ParameterScaling=2^0  OutDataType=sfix(16)  OutScaling=2^0
  Kilim1 : Gain  Gain=30  ParameterDataType=sfix(16)  ParameterScaling=2^0  OutDataType=sfix(16)  OutScaling=2^0
  Kilim2 : Gain  ParameterDataType=sfix(16)  ParameterScaling=2^0  OutDataType=sfix(16)  OutScaling=2^0
  Kilim3 : Gain  ParameterDataType=sfix(16)  ParameterScaling=2^0  OutDataType=sfix(16)  OutScaling=2^0
  Kilim4 : Gain  ParameterDataType=sfix(16)  ParameterScaling=2^0  OutDataType=sfix(16)  OutScaling=2^0
  Kplim : Gain  Gain=3  ParameterDataType=sfix(16)  ParameterScaling=2^0  OutDataType=sfix(16)  OutScaling=2^0
  Kplim1 : Gain  Gain=3  ParameterDataType=sfix(16)  ParameterScaling=2^0  OutDataType=sfix(16)  OutScaling=2^0
  Plimit : Constant  Value=1.0  OutDataType=sfix(16)  OutScaling=2^0
  Plimit1 : Constant  Value=0.0  OutDataType=sfix(16)  OutScaling=2^0
  Saturation1 : Saturate  UpperLimit=pi  LowerLimit=0  OutDataType=fixdt(1, 16)  OutScaling=2^0
  Saturation2 : Saturate  UpperLimit=0  LowerLimit=-pi  OutDataType=fixdt(1, 16)  OutScaling=2^0
  Sum1 : Sum  Inputs=-+|  OutDataType=sfix(16)  OutScaling=2^0
  Sum2 : Sum  Inputs=|++  OutDataType=sfix(16)  OutScaling=2^0
  Sum3 : Sum  OutDataType=sfix(16)  OutScaling=2^0
  Sum4 : Sum  Inputs=|+-  OutDataType=sfix(16)  OutScaling=2^0
  Sum9 : Sum  Inputs=|++  OutDataType=sfix(16)  OutScaling=2^0
  Out1 : Outport
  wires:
  Sum3/1 -> Out1/1
  Saturation2/1 -> Sum3/1
  Saturation1/1 -> Sum3/2
  Sum2/1 -> Saturation1/1
  Integrator2/1 -> Sum2/2
  Kplim1/1 -> Sum2/1
  Kilim1/1 -> Integrator2/1
  Sum1/1 -> Kilim1/1, Kplim1/1
  Sum9/1 -> Saturation2/1
  Integrator1/1 -> Sum9/2
  Kplim/1 -> Sum9/1
  Kilim/1 -> Integrator1/1
  Sum4/1 -> Kilim/1, Kplim/1
  Kilim2/1 -> Sum4/1
  Plimit/1 -> Kilim2/1
  In1/1 -> Kilim3/1
  Kilim3/1 -> Sum4/2, Sum1/1
  Plimit1/1 -> Kilim4/1
  Kilim4/1 -> Sum1/2

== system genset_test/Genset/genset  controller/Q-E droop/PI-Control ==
  In1 : Inport
  Constant1 : Constant  OutDataType=fixdt(1, 16)  OutScaling=2^0
  Gain : Gain  Gain=1000  ParameterDataType=sfix(16)  ParameterScaling=2^0  OutDataType=sfix(16)  OutScaling=2^0
  Gain1 : Gain  Gain=10  ParameterDataType=sfix(16)  ParameterScaling=2^0  OutDataType=sfix(16)  OutScaling=2^0
  Integrator1 : Integrator  InitialCondition=.88  UpperSaturationLimit=1  LowerSaturationLimit=-1
  Sum1 : Sum  Inputs=|++  OutDataType=sfix(16)  OutScaling=2^0
  Sum4 : Sum  Inputs=|++  OutDataType=sfix(16)  OutScaling=2^0
  Out1 : Outport
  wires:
  Gain/1 -> Sum4/1
  Integrator1/1 -> Sum4/2
  In1/1 -> Gain1/1, Gain/1
  Gain1/1 -> Integrator1/1
  Sum1/1 -> Out1/1
  Sum4/1 -> Sum1/1
  Constant1/1 -> Sum1/2

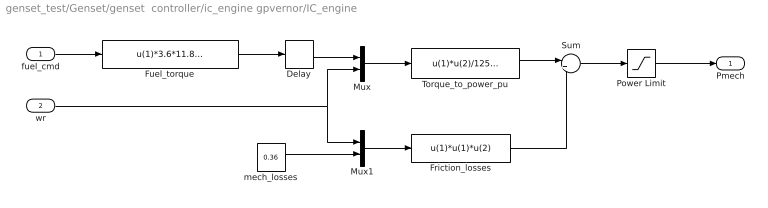
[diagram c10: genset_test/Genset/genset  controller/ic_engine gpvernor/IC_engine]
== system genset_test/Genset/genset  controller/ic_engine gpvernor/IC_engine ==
  fuel_cmd : Inport  OutDataType=fixdt(1, 16)  OutScaling=2^0
  wr : Inport  Port=2  OutDataType=fixdt(1, 16)  OutScaling=2^0
  Delay : TransportDelay  DelayTime=.022
  Friction_losses : Fcn  Expr=u(1)*u(1)*u(2)
  Fuel_torque : Fcn  Expr=u(1)*3.6*11.8238*0.47*1000
  Mux : Mux  Inputs=2
  Mux1 : Mux  Inputs=2
  Power Limit : Saturate  UpperLimit=1  LowerLimit=0  OutDataType=fixdt(1, 16)  OutScaling=2^0
  Sum : Sum  Inputs=|+-  OutDataType=fixdt(1, 16)  OutScaling=2^0
  Torque_to_power_pu : Fcn  Expr=u(1)*u(2)/12500
  mech_losses : Constant  Value=0.36  OutDataType=fixdt(1, 16)  OutScaling=2^0
  Pmech : Outport  OutDataType=fixdt(1, 16)  OutScaling=2^0
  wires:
  Fuel_torque/1 -> Delay/1
  fuel_cmd/1 -> Fuel_torque/1
  Delay/1 -> Mux/1
  wr/1 -> Mux/2, Mux1/1
  mech_losses/1 -> Mux1/2
  Mux1/1 -> Friction_losses/1
  Mux/1 -> Torque_to_power_pu/1
  Torque_to_power_pu/1 -> Sum/1
  Friction_losses/1 -> Sum/2
  Sum/1 -> Power Limit/1
  Power Limit/1 -> Pmech/1

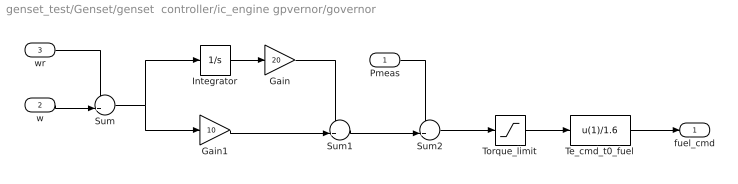
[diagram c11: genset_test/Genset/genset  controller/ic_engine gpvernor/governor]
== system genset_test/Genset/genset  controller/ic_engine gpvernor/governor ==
  Pmeas : Inport  OutDataType=fixdt(1, 16)  OutScaling=2^0
  w : Inport  Port=2  OutDataType=fixdt(1, 16)  OutScaling=2^0
  wr : Inport  Port=3  OutDataType=fixdt(1, 16)  OutScaling=2^0
  Gain : Gain  Gain=20  ParameterDataType=fixdt(1, 16)  ParameterScaling=2^0  OutDataType=fixdt(1, 16)  OutScaling=2^0
  Gain1 : Gain  Gain=10  ParameterDataType=fixdt(1, 16)  ParameterScaling=2^0  OutDataType=fixdt(1, 16)  OutScaling=2^0
  Integrator : Integrator  LimitOutput=on  UpperSaturationLimit=10  LowerSaturationLimit=-10
  Sum : Sum  Inputs=-+|  OutDataType=fixdt(1, 16)  OutScaling=2^0
  Sum1 : Sum  Inputs=++|  OutDataType=fixdt(1, 16)  OutScaling=2^0
  Sum2 : Sum  Inputs=++|  OutDataType=fixdt(1, 16)  OutScaling=2^0
  Te_cmd_t0_fuel : Fcn  Expr=u(1)/1.6
  Torque_limit : Saturate  UpperLimit=1000  LowerLimit=-1000  OutDataType=fixdt(1, 16)  OutScaling=2^0
  fuel_cmd : Outport  OutDataType=fixdt(1, 16)  OutScaling=2^0
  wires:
  w/1 -> Sum/2
  wr/1 -> Sum/1
  Sum/1 -> Integrator/1, Gain1/1
  Integrator/1 -> Gain/1
  Gain/1 -> Sum1/1
  Gain1/1 -> Sum1/2
  Pmeas/1 -> Sum2/1
  Sum1/1 -> Sum2/2
  Sum2/1 -> Torque_limit/1
  Torque_limit/1 -> Te_cmd_t0_fuel/1
  Te_cmd_t0_fuel/1 -> fuel_cmd/1
